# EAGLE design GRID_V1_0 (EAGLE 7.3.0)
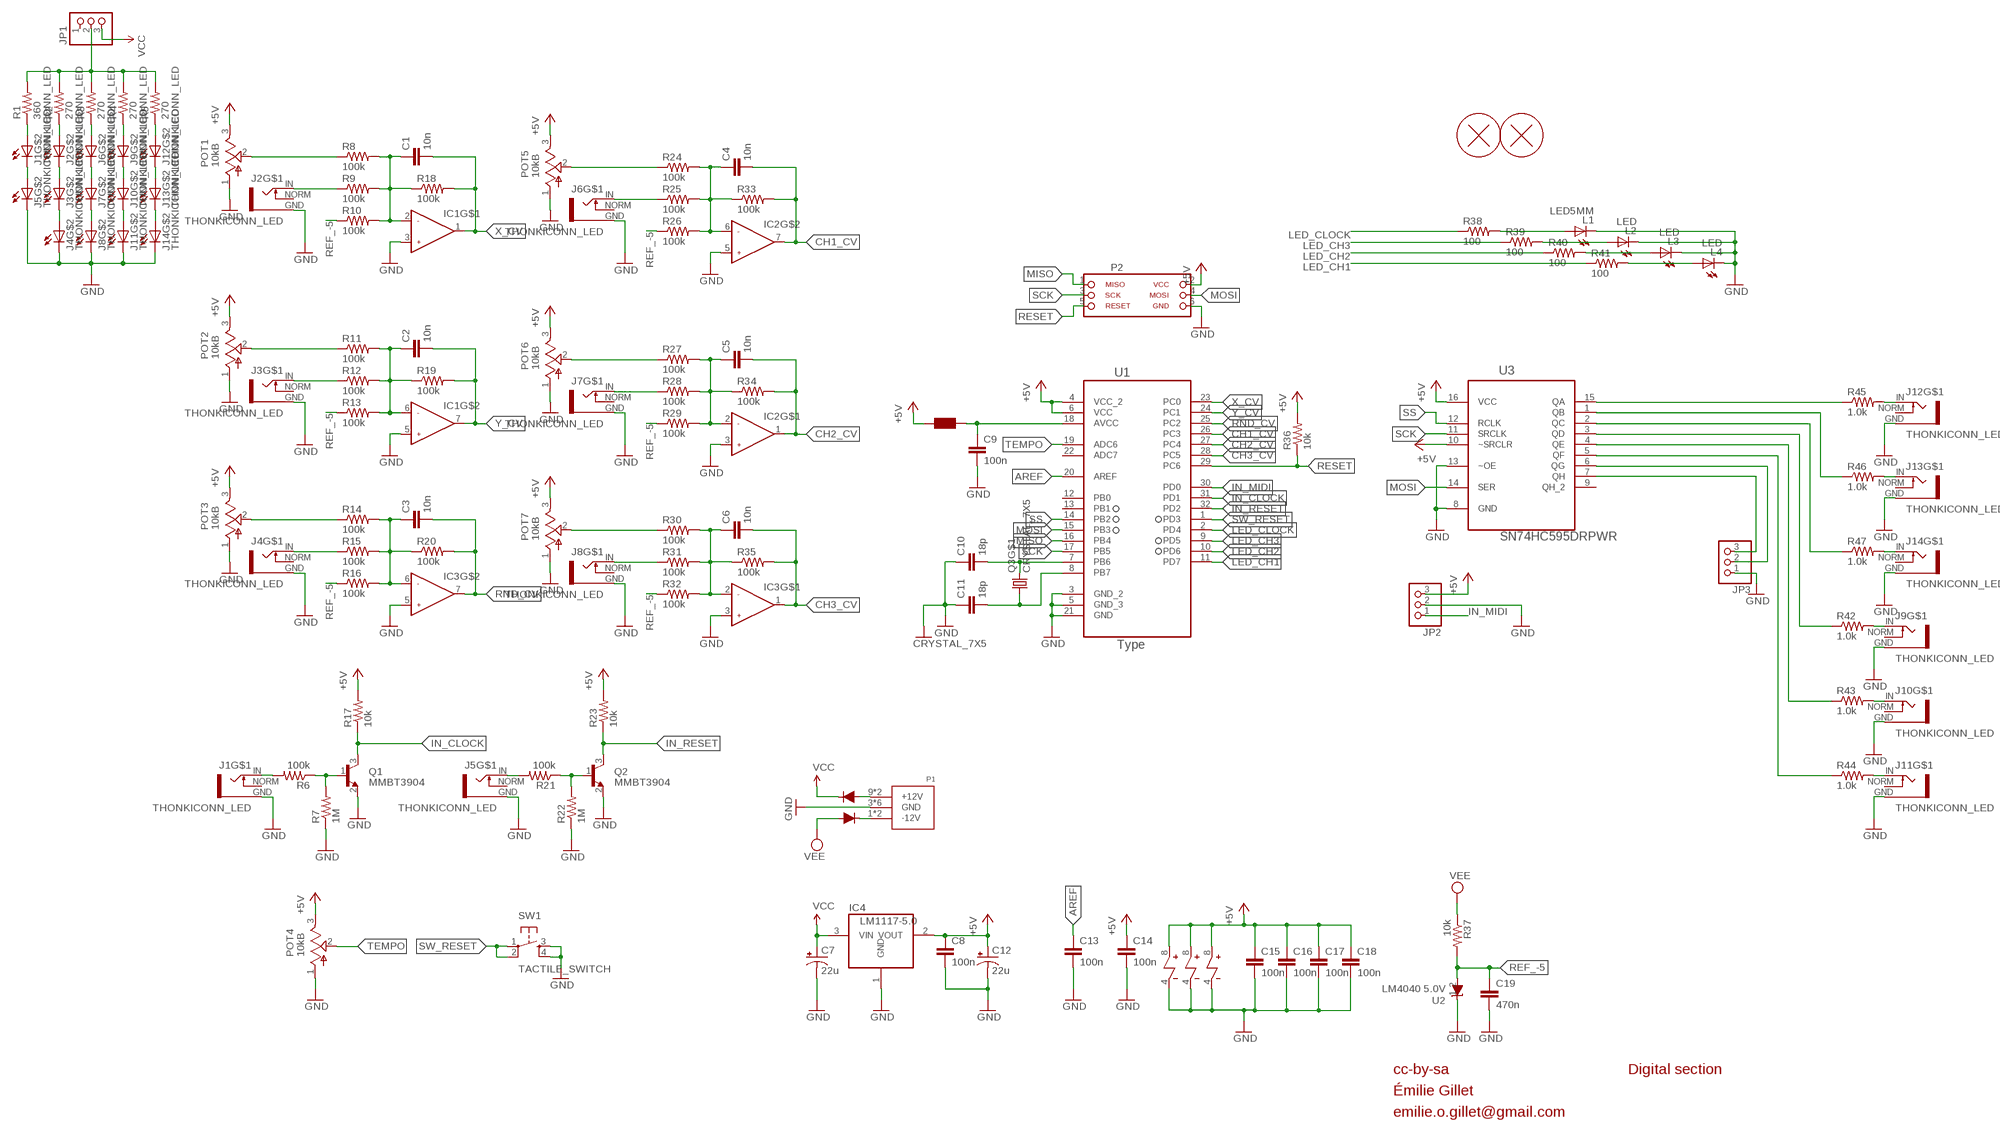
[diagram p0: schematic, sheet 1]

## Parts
C1  10n  CAPACITOR  [RESISTOR_0603]
C2  10n  CAPACITOR  [RESISTOR_0603]
C3  10n  CAPACITOR  [RESISTOR_0603]
C4  10n  CAPACITOR  [RESISTOR_0603]
C5  10n  CAPACITOR  [RESISTOR_0603]
C6  10n  CAPACITOR  [RESISTOR_0603]
C7  22u  CAP_POLC  [PANASONIC_C]
C8  100n  CAPACITOR  [RESISTOR_0603]
C9  100n  CAPACITOR  [RESISTOR_0603]
C10  18p  CAPACITOR  [RESISTOR_0603]
C11  18p  CAPACITOR  [RESISTOR_0603]
C12  22u  CAP_POLC  [PANASONIC_C]
C13  100n  CAPACITOR  [RESISTOR_0603]
C14  100n  CAPACITOR  [RESISTOR_0603]
C15  100n  CAPACITOR  [RESISTOR_0603]
C16  100n  CAPACITOR  [RESISTOR_0603]
C17  100n  CAPACITOR  [RESISTOR_0603]
C18  100n  CAPACITOR  [RESISTOR_0603]
C19  470n  CAPACITOR  [RESISTOR_0603]
D1  1N5819HW  DIODE  [SOD123]
D2  1N5819HW  DIODE  [SOD123]
F1  FERRITE-BEAD  [RESISTOR_0603]
H1  PCB_SCREW  [PCB_SCREW]
H2  PCB_SCREW  [PCB_SCREW]
IC1  OPAMP_DUAL  [SOIC8]
IC2  OPAMP_DUAL  [SOIC8]
IC3  OPAMP_DUAL  [SOIC8]
IC4  LM1117-5.0  REG1117  [SOT223]
J1  THONKICONN_LED  [LED_JACK]
J2  THONKICONN_LED  [LED_JACK]
J3  THONKICONN_LED  [LED_JACK]
J4  THONKICONN_LED  [LED_JACK]
J5  THONKICONN_LED  [LED_JACK]
J6  THONKICONN_LED  [LED_JACK]
J7  THONKICONN_LED  [LED_JACK]
J8  THONKICONN_LED  [LED_JACK]
J9  THONKICONN_LED  [LED_JACK]
J10  THONKICONN_LED  [LED_JACK]
J11  THONKICONN_LED  [LED_JACK]
J12  THONKICONN_LED  [LED_JACK]
J13  THONKICONN_LED  [LED_JACK]
J14  THONKICONN_LED  [LED_JACK]
JP1  PINHD-1X3  [1X03]
JP2  PINHD-1X3  [1X03]
JP3  PINHD-1X3  [1X03]
L1  LED5MM  [LED_5MM]
L2  LED  [LED_3MM]
L3  LED  [LED_3MM]
L4  LED  [LED_3MM]
P1  POWER_SIMPLE10  [POWER_10]
P2  PINHD-SPI  [2X03]
POT1  10kB  POT_VERTICAL  [ALPS_POT_VERTICAL]
POT2  10kB  POT_VERTICAL  [ALPS_POT_VERTICAL]
POT3  10kB  POT_VERTICAL  [ALPS_POT_VERTICAL]
POT4  10kB  POT_VERTICAL  [ALPS_POT_VERTICAL]
POT5  10kB  POT_VERTICAL  [ALPS_POT_VERTICAL]
POT6  10kB  POT_VERTICAL  [ALPS_POT_VERTICAL]
POT7  10kB  POT_VERTICAL  [ALPS_POT_VERTICAL]
Q1  MMBT3904  MMBT3904SOT23  [SOT23]
Q2  MMBT3904  MMBT3904SOT23  [SOT23]
Q3  CRYSTAL_7X5  [7X5_CRYSTAL]
R1  360  RESISTOR  [RESISTOR_0603]
R2  270  RESISTOR  [RESISTOR_0603]
R3  270  RESISTOR  [RESISTOR_0603]
R4  270  RESISTOR  [RESISTOR_0603]
R5  270  RESISTOR  [RESISTOR_0603]
R6  100k  RESISTOR  [RESISTOR_0603]
R7  1M  RESISTOR  [RESISTOR_0603]
R8  100k  RESISTOR  [RESISTOR_0603]
R9  100k  RESISTOR  [RESISTOR_0603]
R10  100k  RESISTOR  [RESISTOR_0603]
R11  100k  RESISTOR  [RESISTOR_0603]
R12  100k  RESISTOR  [RESISTOR_0603]
R13  100k  RESISTOR  [RESISTOR_0603]
R14  100k  RESISTOR  [RESISTOR_0603]
R15  100k  RESISTOR  [RESISTOR_0603]
R16  100k  RESISTOR  [RESISTOR_0603]
R17  10k  RESISTOR  [RESISTOR_0603]
R18  100k  RESISTOR  [RESISTOR_0603]
R19  100k  RESISTOR  [RESISTOR_0603]
R20  100k  RESISTOR  [RESISTOR_0603]
R21  100k  RESISTOR  [RESISTOR_0603]
R22  1M  RESISTOR  [RESISTOR_0603]
R23  10k  RESISTOR  [RESISTOR_0603]
R24  100k  RESISTOR  [RESISTOR_0603]
R25  100k  RESISTOR  [RESISTOR_0603]
R26  100k  RESISTOR  [RESISTOR_0603]
R27  100k  RESISTOR  [RESISTOR_0603]
R28  100k  RESISTOR  [RESISTOR_0603]
R29  100k  RESISTOR  [RESISTOR_0603]
R30  100k  RESISTOR  [RESISTOR_0603]
R31  100k  RESISTOR  [RESISTOR_0603]
R32  100k  RESISTOR  [RESISTOR_0603]
R33  100k  RESISTOR  [RESISTOR_0603]
R34  100k  RESISTOR  [RESISTOR_0603]
R35  100k  RESISTOR  [RESISTOR_0603]
R36  10k  RESISTOR  [RESISTOR_0603]
R37  10k  RESISTOR  [RESISTOR_0603]
R38  100  RESISTOR  [RESISTOR_0603]
R39  100  RESISTOR  [RESISTOR_0603]
R40  100  RESISTOR  [RESISTOR_0603]
R41  100  RESISTOR  [RESISTOR_0603]
R42  1.0k  RESISTOR  [RESISTOR_0603]
R43  1.0k  RESISTOR  [RESISTOR_0603]
R44  1.0k  RESISTOR  [RESISTOR_0603]
R45  1.0k  RESISTOR  [RESISTOR_0603]
R46  1.0k  RESISTOR  [RESISTOR_0603]
R47  1.0k  RESISTOR  [RESISTOR_0603]
SW1  TACTILE_SWITCH  [TACTILE-PTH]
U1  ATMEGA328P-AU  [QFP80P900X900X120-32N]
U2  LM4040 5.0V  LM4040SOT23  [SOT23]
U3  SN74HC595DRPWR  [TSSOP16]

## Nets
+5V [wide]: C8.1 C12.+ C14.1 C15.1 C16.1 C17.1 C18.1 F1.2 IC1.8 IC2.8 IC3.8 IC4.2(VOUT) JP2.3 P2.2 POT1.3(B) POT2.3(B) POT3.3(B) POT4.3(B) POT5.3(B) POT6.3(B) POT7.3(B) R17.2 R23.2 R36.2 U1.4(VCC_2) U1.6(VCC) U3.10(~SRCLR) U3.16(VCC)
AREF: C13.1 U1.20(AREF)
CH1_CV: C4.2 IC2.7 R33.2 U1.26(PC3)
CH2_CV: C5.2 IC2.1 R34.2 U1.27(PC4)
CH3_CV: C6.2 IC3.1 R35.2 U1.28(PC5)
CLOCK_OUT: JP3.2 U3.6(QG)
GATE1_IN: J1.IN R6.2
GATE1_LED: L1.A R38.2
GATE2_IN: J5.IN R21.2
GATE2_LED: L2.A R39.2
GATE3_LED: L3.A R40.2
GATE4_LED: L4.A R41.2
GND: C7.- C8.2 C9.2 C10.1 C11.1 C12.- C13.2 C14.2 C15.2 C16.2 C17.2 C18.2 C19.2 IC1.3 IC1.4 IC1.5 IC2.3 IC2.4 IC2.5 IC3.3 IC3.4 IC3.5 IC4.1(GND) J1.GND J2.GND J3.GND J4.C J4.GND J5.C J5.GND J6.GND J7.GND J8.C J8.GND J9.GND J10.GND J11.C J11.GND J12.GND J13.GND J14.C J14.GND JP2.2 JP3.1 L1.K(C) L2.K(C) L3.K(C) L4.K(C) P1.3(GND) P1.4(GND) P1.5(GND) P1.6(GND) P1.7(GND) P1.8(GND) P2.6 POT1.1(A) POT2.1(A) POT3.1(A) POT4.1(A) POT5.1(A) POT6.1(A) POT7.1(A) Q1.2(E) Q2.2(E) Q3.2(GND) Q3.4(GND) R7.1 R22.1 SW1.3 SW1.4 U1.3(GND_2) U1.5(GND_3) U1.21(GND) U2.1(C) U3.8(GND) U3.13(~OE)
IN_CLOCK: Q1.3(C) R17.1 U1.31(PD1)
IN_MIDI: JP2.1 U1.30(PD0)
IN_RESET: Q2.3(C) R23.1 U1.32(PD2)
LED_CH1: R41.1 U1.11(PD7)
LED_CH2: R40.1 U1.10(PD6)
LED_CH3: R39.1 U1.9(PD5)
LED_CLOCK: R38.1 U1.2(PD4)
MISO: P2.1 U1.16(PB4)
MOSI: P2.4 U1.15(PB3) U3.14(SER)
N$1: Q1.1(B) R6.1 R7.2
N$2: Q2.1(B) R21.1 R22.2
N$3 [wide]: D1.+ P1.9(+12V) P1.10(+12V)
N$4: J11.IN R44.2
N$5: J10.IN R43.2
N$6: J9.IN R42.2
N$8: J2.C J3.A
N$9: POT1.2(W) R8.1
N$10: J2.IN R9.1
N$11: J3.C J4.A
N$12: C2.1 IC1.6 R11.2 R12.2 R13.2 R19.1
N$13: POT2.2(W) R11.1
N$14: J3.IN R12.1
N$15: C3.1 IC3.6 R14.2 R15.2 R16.2 R20.1
N$16: POT3.2(W) R14.1
N$17: J4.IN R15.1
N$18: C4.1 IC2.6 R24.2 R25.2 R26.2 R33.1
N$19: POT5.2(W) R24.1
N$20: J6.IN R25.1
N$21: C5.1 IC2.2 R27.2 R28.2 R29.2 R34.1
N$22: POT6.2(W) R27.1
N$23: J7.IN R28.1
N$24: C6.1 IC3.2 R30.2 R31.2 R32.2 R35.1
N$25: POT7.2(W) R30.1
N$26: J8.IN R31.1
N$27: R45.1 U3.15(QA)
N$28: R46.1 U3.1(QB)
N$29: C1.1 IC1.2 R8.2 R9.2 R10.2 R18.1
N$30: R47.1 U3.2(QC)
N$31: R42.1 U3.3(QD)
N$32: R43.1 U3.4(QE)
N$33: R44.1 U3.5(QF)
N$34: J12.IN R45.2
N$35: J13.IN R46.2
N$36: J14.IN R47.2
N$37: J7.C J8.A
N$38: J6.C J7.A
N$39: C9.1 F1.1 U1.18(AVCC)
N$40: J9.C J10.A
N$41: J10.C J11.A
N$42: J12.C J13.A
N$43: J13.C J14.A
N$44: J12.A R5.1
N$45: J9.A R4.1
N$46: J6.A R3.1
N$47: J2.A R2.1
N$48: J1.A R1.1
N$49: J1.C J5.A
N$50 [wide]: JP1.2 R1.2 R2.2 R3.2 R4.2 R5.2
N$51 [wide]: D2.- P1.1(-12V) P1.2(-12V)
N$82: C11.2 Q3.1 U1.8(PB7)
N$83: C10.2 Q3.3 U1.7(PB6)
RANDOM_GATE: JP3.3 U3.7(QH)
REF_-5: C19.1 R10.1 R13.1 R16.1 R26.1 R29.1 R32.1 R37.2 U2.2(A)
RESET: P2.5 R36.1 U1.29(PC6)
RND_CV: C3.2 IC3.7 R20.2 U1.25(PC2)
SCK: P2.3 U1.17(PB5) U3.11(SRCLK)
SS: U1.14(PB2) U3.12(RCLK)
SW_RESET: SW1.1 SW1.2 U1.1(PD3)
TEMPO: POT4.2(W) U1.19(ADC6)
VCC [wide]: C7.+ D1.- IC4.3(VIN) JP1.3
VEE [wide]: D2.+ R37.1
X_CV: C1.2 IC1.1 R18.2 U1.23(PC0)
Y_CV: C2.2 IC1.7 R19.2 U1.24(PC1)
Unconnected: J1.NORM J2.NORM J3.NORM J4.NORM J5.NORM J6.NORM J7.NORM J8.NORM J9.NORM J10.NORM J11.NORM J12.NORM J13.NORM J14.NORM JP1.1 U1.12(PB0) U1.13(PB1) U1.22(ADC7) U3.9(QH_2)

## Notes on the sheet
- cc-by-sa | Digital section
- Émilie Gillet
- emilie.o.gillet@gmail.com

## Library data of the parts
C1-C6 C8-C11 C13-C19 = parts_aman:CAPACITOR
C7 C12 = parts_aman:CAP_POL
D1 D2 = parts_aman:DIODE
F1 = parts_aman:FERRITE-BEAD
H1 H2 = parts_aman:PCB_SCREW
IC1-IC3 = parts_aman:OPAMP_DUAL
IC4 = og-vreg:REG1117: 800mA and 1A Low Dropout (LDO) Positive Regulator 1.8V, 2.5V, 2.85V, 3.3V, 5V, and Adj
J1-J14 = parts_aman:THONKICONN_LED
JP1-JP3 = parts_aman:PINHD-1X3: PIN HEADER
L1-L4 = parts_aman:LED
P1 = parts_aman:POWER_SIMPLE
P2 = parts_aman:PINHD-SPI: PIN HEADER
POT1-POT7 = parts_aman:POT_VERTICAL
Q1 Q2 = parts_aman:MMBT3904
Q3 = parts_aman:CRYSTAL_7X5
R1-R47 = parts_aman:RESISTOR
SW1 = parts_aman:TACTILE_SWITCH
U1 = parts_aman:ATMEGA328P-AU; DESCRIPTION: 8-bit Microcontroller with In-System Programmable Flash; MPN: ATMEGA328P-AU; OC_FARNELL: 1715486; OC_NEWARK: 14R4631; PACKAGE: TQFP-32; SUPPLIER: Atmel
U2 = parts_aman:LM4040
U3 = parts_aman:SN74HC595DR: 8-BIT SHIFT REGISTERS WITH 3-STATE OUTPUT REGISTERS

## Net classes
0 default: width 0.152 mm, drill 0.305 mm, clearance 0.152 mm
1 wide: width 0.305 mm, drill 0.305 mm, clearance 0.152 mm

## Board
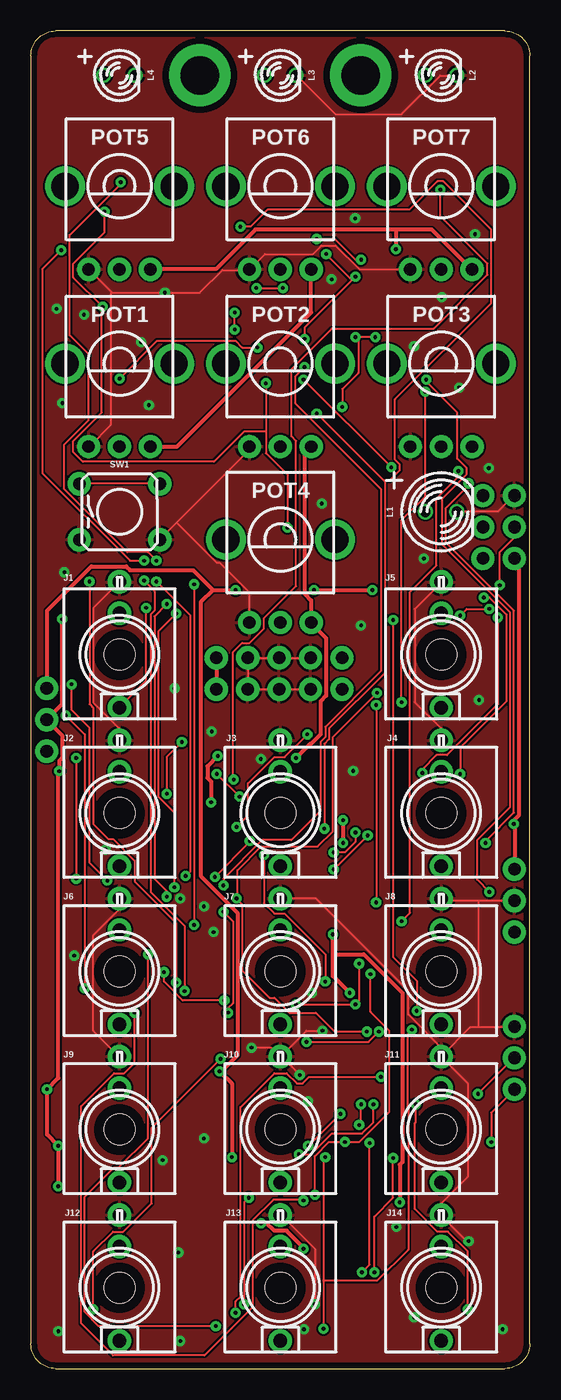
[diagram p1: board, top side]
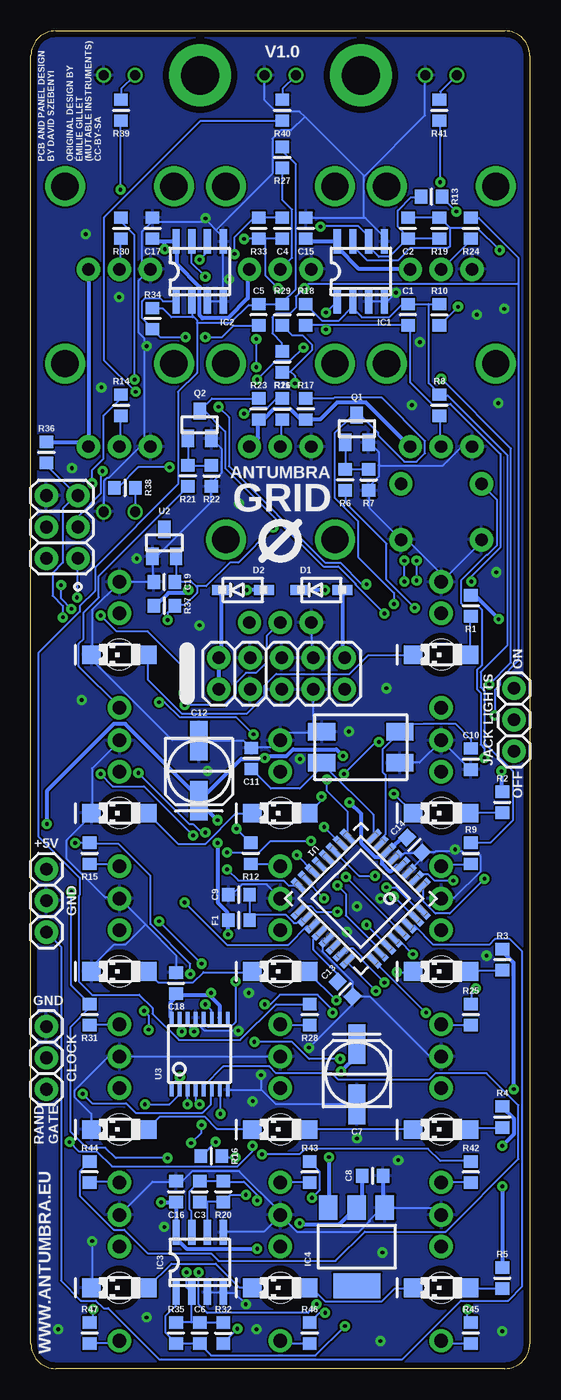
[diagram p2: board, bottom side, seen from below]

Size 40.3 x 108 mm. Coordinates in mm from the lower left corner, seen from the top.
Outline: 2,0 38.3,0 arc90 40.3,2 40.3,106 arc90 38.3,108 2,108 arc90 0,106 0,2 arc90 2,0
Copper layers (1*16): Top 0.035mm / dielectric 1.5mm / Bottom 0.035mm
Design rules "PCBCart-Standard": minimum track width 6mil, minimum drill 12mil, track to track 6mil, track to pad 6mil, pad to pad 6mil, via to via 6mil, smd to smd 6mil, copper to edge 20mil, drill to drill 8mil, minimum pad ring 8mil, minimum via ring 10mil, stop-mask expansion 3mil, vias tented up to drill 25mil, thermal gap 8mil

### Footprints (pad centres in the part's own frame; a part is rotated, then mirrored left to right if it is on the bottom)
RESISTOR_0603 = smd 1 x 1.1: 1 -0.85,0; 2 0.85,0
PANASONIC_C = smd 3.2 x 1.4: + 2.378,0; - -2.478,0
SOD123 = smd 1.6 x 0.8: + 1.7,0; - -1.7,0
PCB_SCREW = drill 3.1 pad 5: P$1 0,0
SOIC8 = smd 0.6 x 2: 1 -1.905,-2.419; 2 -0.635,-2.419; 3 0.635,-2.419; 4 1.905,-2.419; 5 1.905,2.42; 6 0.635,2.42; 7 -0.635,2.42; 8 -1.905,2.42
SOT223 = smd 1.499 x 2.007: 1 -2.261,-3.15; 2 0.025,-3.15; 3 2.311,-3.15 | smd 3.81 x 2.007: 4 0,3.15
LED_JACK = smd 1.5 x 1.5 bottom: A 2.266,0; C -2.266,0 | drill 1.1 pad 1.88: GND 0,-5.88; IN 0,4.28; NORM 0,-3.34 | hole 2.5: 0,0
1X03 = drill 1.016 pad 1.88: 1 -2.54,0; 2 0,0; 3 2.54,0
LED_5MM = drill 0.813: A -1.27,0; K 1.27,0
LED_3MM = drill 0.813: A -1.27,0; K 1.27,0
POWER_10 = drill 1.016 pad 1.88: 1 -5.08,-1.27; 2 -5.08,1.27; 3 -2.54,-1.27; 4 -2.54,1.27; 5 0,-1.27; 6 0,1.27; 7 2.54,-1.27; 8 2.54,1.27; 9 5.08,-1.27; 10 5.08,1.27
2X03 = drill 1.016 pad 1.88: 1 -2.54,-1.27; 2 -2.54,1.27; 3 0,-1.27; 4 0,1.27; 5 2.54,-1.27; 6 2.54,1.27
ALPS_POT_VERTICAL = drill 1 pad 1.88: 1 -2.5,-6.7; 2 0,-6.7; 3 2.5,-6.7 | drill 2.2 pad 3.175: P$4 4.4,0; P$5 -4.4,0
SOT23 = smd 1 x 1.4: 1 -0.95,-1.1; 2 0.95,-1.1; 3 0,1.1
7X5_CRYSTAL = smd 2.2 x 1.4: 1 -3.15,-1.25; 2 -3.15,1.25; 3 3.15,1.25; 4 3.15,-1.25
TACTILE-PTH = drill 1.016 pad 1.88: 1 -3.251,2.261; 2 3.251,2.261; 3 -3.251,-2.261; 4 3.251,-2.261
QFP80P900X900X120-32N = smd 1.473 x 0.508: 1 -4.242,2.794; 2 -4.242,2.007; 3 -4.242,1.194; 4 -4.242,0.406; 5 -4.242,-0.406; 6 -4.242,-1.194; 7 -4.242,-2.007; 8 -4.242,-2.794; 17 4.242,-2.794; 18 4.242,-2.007; 19 4.242,-1.194; 20 4.242,-0.406; 21 4.242,0.406; 22 4.242,1.194; 23 4.242,2.007; 24 4.242,2.794 | smd 0.508 x 1.473: 9 -2.794,-4.242; 10 -2.007,-4.242; 11 -1.194,-4.242; 12 -0.406,-4.242; 13 0.406,-4.242; 14 1.194,-4.242; 15 2.007,-4.242; 16 2.794,-4.242; 25 2.794,4.242; 26 2.007,4.242; 27 1.194,4.242; 28 0.406,4.242; 29 -0.406,4.242; 30 -1.194,4.242; 31 -2.007,4.242; 32 -2.794,4.242
TSSOP16 = smd 0.305 x 0.991: 1 -2.275,-2.918; 2 -1.625,-2.918; 3 -0.975,-2.918; 4 -0.325,-2.918; 5 0.325,-2.918; 6 0.975,-2.918; 7 1.625,-2.918; 8 2.275,-2.918; 9 2.275,2.918; 10 1.625,2.918; 11 0.975,2.918; 12 0.325,2.918; 13 -0.325,2.918; 14 -0.975,2.918; 15 -1.625,2.918; 16 -2.275,2.918

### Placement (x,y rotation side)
C1  9.84,85.09 270 bottom
C2  9.84,92.08 90 bottom
C3  26.67,14.29 90 bottom
C4  20,92.08 90 bottom
C5  21.91,85.09 270 bottom
C6  26.67,2.86 270 bottom
C7  13.97,23.81 90 bottom
C8  12.7,15.56 0 bottom
C9  23.5,38.26 180 bottom
C10  4.76,49.21 90 bottom
C11  22.49,49.26 270 bottom
C12  26.73,48.21 270 bottom
C13  14.92,30.64 315 bottom
C14  9.32,42.27 315 bottom
C15  18.1,92.08 90 bottom
C16  28.57,14.29 90 bottom
C17  30.48,92.08 90 bottom
C18  28.57,31.11 90 bottom
C19  29.53,63.5 180 bottom
D1  16.83,62.87 0 bottom
D2  23.18,62.87 0 bottom
F1  23.5,36.2 180 bottom
H1  13.64,104.42 0 top
H2  26.64,104.42 0 top
IC1  13.65,88.58 0 bottom
IC2  26.67,88.58 0 bottom
IC3  26.67,8.57 0 bottom
IC4  13.97,9.84 180 bottom
J1  7.16,57.64 180 top
J2  7.16,44.85 180 top
J3  20.15,44.85 180 top
J4  33.15,44.85 180 top
J5  33.15,57.64 180 top
J6  7.16,32.07 180 top
J7  20.15,32.07 180 top
J8  33.15,32.07 180 top
J9  7.16,19.31 180 top
J10  20.15,19.31 180 top
J11  33.15,19.31 180 top
J12  7.16,6.52 180 top
J13  20.15,6.52 180 top
J14  33.15,6.52 180 top
JP1  1.27,52.39 90 bottom
JP2  39.05,37.78 90 bottom
JP3  39.05,25.08 270 bottom
L1  33.15,69.18 0 top
L2  33.15,104.42 0 top
L3  20.15,104.42 0 top
L4  7.16,104.42 0 top
P1  20.05,56.11 0 bottom
P2  37.78,67.94 90 bottom
POT1  7.16,81.14 0 top
POT2  20.15,81.14 0 top
POT3  33.15,81.14 0 top
POT4  20.15,66.94 0 top
POT5  7.16,95.46 0 top
POT6  20.15,95.46 0 top
POT7  33.15,95.46 0 top
Q1  13.97,75.88 0 bottom
Q2  26.67,76.2 0 bottom
Q3  13.65,50.16 0 bottom
R1  4.76,61.59 90 bottom
R2  2.22,45.72 90 bottom
R3  2.22,33.02 90 bottom
R4  2.22,20.32 90 bottom
R5  2.22,7.3 90 bottom
R6  14.92,71.75 270 bottom
R7  13.02,71.75 90 bottom
R8  7.3,77.79 90 bottom
R9  4.76,41.59 90 bottom
R10  7.3,85.09 90 bottom
R11  20,77.47 90 bottom
R12  22.54,41.59 90 bottom
R13  7.94,94.61 180 bottom
R14  33.02,77.79 90 bottom
R15  35.56,41.59 90 bottom
R16  25.72,17.14 180 bottom
R17  18.1,77.47 270 bottom
R18  18.1,85.09 270 bottom
R19  7.3,92.08 90 bottom
R20  24.77,14.29 90 bottom
R21  27.62,72.07 270 bottom
R22  25.72,72.07 90 bottom
R23  21.91,77.47 270 bottom
R24  4.76,92.08 90 bottom
R25  4.76,28.57 90 bottom
R26  20,81.28 90 bottom
R27  20,97.79 90 bottom
R28  17.78,28.57 90 bottom
R29  20,85.09 90 bottom
R30  33.02,92.08 90 bottom
R31  35.56,28.57 90 bottom
R32  24.77,2.86 90 bottom
R33  21.91,92.08 90 bottom
R34  30.48,84.77 270 bottom
R35  28.57,2.86 270 bottom
R36  39.05,73.98 90 bottom
R37  29.53,61.59 0 bottom
R38  32.7,71.12 0 bottom
R39  33.02,101.6 90 bottom
R40  20,101.6 90 bottom
R41  7.3,101.6 90 bottom
R42  4.76,15.88 270 bottom
R43  17.78,15.88 270 bottom
R44  35.56,15.88 270 bottom
R45  4.76,2.86 270 bottom
R46  17.78,2.86 270 bottom
R47  35.56,2.86 270 bottom
SW1  7.16,69.18 0 top
U1  13.65,37.94 225 bottom
U2  29.53,66.67 0 bottom
U3  26.67,25.4 0 bottom
U$1  [LOGO_3.5]  20.16,66.83 0 bottom

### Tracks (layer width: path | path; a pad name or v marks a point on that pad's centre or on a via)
+5V  (via drill 0.3)
  Top 0.305: 29.49,91.97 32.38,91.97 35.59,88.77 POT7.3 | 29.49,91.97 18.14,91.97 14.94,88.77 9.68,88.77 POT5.3 | 29.49,91.97 v29.49,90.37 | 24.38,33.45 24.38,31.7 v25.76,30.33 | 24.38,33.45 v24.38,35.05 | v29.79,13.41 29.79,16.46 30.02,16.69 30.02,30.33 26.9,33.45 24.38,33.45 | v18.59,11.73 19.05,11.73 19.66,11.12 20.65,11.12 22.02,9.75 v22.02,9.68 | 39.09,43.97 39.09,44.35 39.4,44.65 39.4,65.08 39.09,65.38 P2.2 | 39.09,43.97 39.09,40.39 JP2.3 | v14.55,45.72 14.55,47.4 14.25,47.7 14.25,48.62 v15.09,49.45 | POT2.3 22.63,74.37 22.1,73.84 22.1,62.56 22.63,62.03 22.63,60.27 POT4.3 22.71,60.12 23.85,58.98 23.85,54.33 23.39,53.87 23.39,51.21 22.63,50.44 22.55,50.44 v21.41,49.3 | v39.01,43.97 39.09,43.97 | v25.22,44.27 v25.22,42.44 | POT6.3 22.63,88.7 22.63,85.27 11.81,74.45 9.68,74.45 POT1.3
  Bottom 0.305: C14.1 10.25,42.88 U1.6 | C8.1 13.55,13.44 IC4.2 14.1,12.95 15.39,11.66 18.52,11.66 v18.59,11.73 | U3.16 29.05,28.42 29.05,29.53 28.57,30 C18.1 28.5,30.18 25.91,30.18 | 29.49,91 IC2.8 28.5,90.91 28.5,89.15 26.67,87.33 26.67,85.04 26.44,84.81 24.38,84.81 22.78,86.41 22.78,88.62 22.71,88.7 POT6.3 | 29.49,91 30.26,91 C17.1 | C15.1 17.88,91 IC1.8 15.47,90.91 15.47,90.45 13.79,88.77 9.68,88.77 POT5.3 | R36.2 39.01,74.75 35.97,74.75 35.66,74.45 POT3.3 35.89,74.83 35.59,75.13 35.59,88.7 POT7.3 | v29.49,90.37 29.49,91 | 25.91,30.18 25.07,29.34 25.07,28.35 U3.10 | v24.38,35.05 24.38,36.2 F1.2 24.46,36.27 24.46,36.88 25.22,37.64 v25.22,42.44 | v25.76,30.33 25.91,30.18 | v29.79,13.41 28.65,13.41 C16.1 IC3.8 28.5,10.9 28.5,10.44 27.74,9.68 v22.02,9.68 | U1.4 10.44,40.62 10.74,40.62 11.2,40.16 11.35,40.16 11.96,40.77 11.96,41.3 11.58,41.68 U1.6 | v14.55,45.72 13.64,44.81 13.64,42.44 12.5,41.3 12.04,41.3 U1.6 | v15.09,49.45 15.62,49.99 19.13,49.99 19.66,49.45 21.41,49.45 | 21.41,49.45 21.64,49.45 21.87,49.23 23.32,49.23 26.67,45.87 C12.+ | POT2.3 22.63,74.45 21.95,75.13 21.95,76.5 R23.2 21.87,76.66 21.49,76.66 20.65,77.5 19.36,77.5 18.52,76.66 18.14,76.66 R17.2 17.98,76.66 16.92,76.66 15.54,78.03 13.26,78.03 9.68,74.45 POT1.3 | v21.41,49.3 21.41,49.45 | v39.01,43.97 39.01,46.63 33.6,52.05 32.69,52.05 26.67,46.02 C12.+ | v25.22,44.27 26.67,45.72 C12.+
AREF
  Bottom 0.152: C13.1 15.52,31.88 17.46,33.81 17.46,34.71 U1.20
CH1_CV  (via drill 0.3)
  Top 0.152: v15.54,39.01 15.54,39.55 18.67,42.67 21.03,42.67 23.39,45.03 23.39,50.6 23.77,50.98 23.77,51.82 28.27,56.31 28.27,71.02 21.34,77.95 21.34,80.09 v22.1,80.85 | v22.1,83.13 22.1,84.05 v26.21,88.16 25.91,87.94 v23.85,89.99
  Bottom 0.152: C4.2 20.04,92.96 21.87,92.96 R33.2 21.95,92.89 22.33,92.89 23.85,91.36 v23.85,89.99 | v15.54,39.01 14.86,38.33 14.86,36.58 12.12,33.83 12.12,33.53 U1.26 | v22.1,83.13 v22.1,80.85 | v26.21,88.16 27.36,89.31 27.36,90.98 IC2.7
CH2_CV  (via drill 0.3)
  Top 0.152: v27.81,83.29 26.44,83.29 | v13.18,63.32 v13.18,35.81 | v25.15,77.65 25.15,79.1 26.44,80.39 26.44,83.29 | 26.44,83.29 v26.21,83.29
  Bottom 0.152: v26.21,83.29 24.84,83.29 23.93,84.2 21.95,84.2 C5.2 | v27.81,83.29 29.87,83.29 30.48,83.9 R34.2 30.48,83.97 31.32,84.81 31.32,86.18 31.09,86.41 29.87,86.41 29.64,86.18 28.57,86.18 IC2.1 | v13.18,35.81 11.51,34.14 U1.27 | v13.18,63.32 13.56,63.32 15.32,65.08 16.54,65.08 24.31,72.85 24.31,76.81 v25.15,77.65
CH3_CV  (via drill 0.3)
  Top 0.152: v9.45,33.45 9.45,18.59 7.09,16.23 6.71,16.23 4.34,13.87 4.34,4.57 5.49,3.43 v14.94,3.43
  Bottom 0.152: 28.57,2.06 26.67,2.06 C6.2 26.67,1.98 25.76,1.07 17.3,1.07 v14.94,3.43 | v9.45,33.45 10.59,34.59 10.9,34.59 U1.28 | IC3.1 28.57,5.11 29.41,4.27 29.41,2.9 28.57,2.06 | 28.57,2.06 R35.2
CLOCK_OUT  (via drill 0.3)
  Top 0.152: v36.12,22.17 39.01,25.07 JP3.2
  Bottom 0.152: v36.12,22.17 35.36,21.41 32.61,21.41 31.85,20.65 26.44,20.65 25.76,21.34 25.76,22.48 U3.6
GATE1_IN  (via drill 0.3)
  Top 0.152: v9.3,61.42 9.3,55.55 7.16,53.42 J1.IN
  Bottom 0.152: v9.3,61.42 11.58,63.7 11.58,66.6 14.86,69.88 14.86,70.87 R6.2
GATE1_LED
  Bottom 0.152: R38.2 31.85,71.09 31.85,69.19 L1.A
GATE2_IN
  Bottom 0.152: R21.2 27.66,71.17 34.82,64.01 34.82,62.26 36.04,61.04 36.04,58.9 36.42,58.52 36.42,56.69 33.15,53.42 J5.IN
GATE2_LED
  Bottom 0.152: R39.2 32.99,102.49 32.99,103.33 31.93,104.39 L2.A
GATE3_LED
  Bottom 0.152: R40.2 19.96,102.49 19.96,103.33 18.9,104.39 L3.A
GATE4_LED
  Bottom 0.152: R41.2 7.24,102.49 7.24,103.1 5.94,104.39 L4.A
GND  (via drill 0.3)
  Top 0.152: v35.36,10.29 35.2,10.29 33.15,12.34 J14.GND 33.15,13.34 35.28,15.47 35.28,23.01 33.15,25.15 J11.GND | v22.94,5.18 22.94,9.68 20.19,12.42 J13.GND | 36.2,37.8 33.3,37.8 J8.GND | 36.2,37.8 39.01,37.8 JP2.2 | J6.GND 7.09,37.95 7.09,37.03 5.03,34.98 5.03,27.28 7.09,25.22 J9.GND | v23.55,27.28 22.25,27.28 20.19,25.22 | 36.2,27.58 35.51,27.58 33.15,25.22 J11.GND | 36.2,27.58 39.01,27.58 JP3.1 | J7.GND 20.19,37.95 23.01,37.95 30.48,30.48 30.48,28.57 33.45,25.6 J11.GND | 20.19,25.22 v21.72,23.7 | 20.19,25.22 J10.GND 20.12,25.22 19.43,25.91 v17.83,25.91 | 36.2,27.58 36.2,37.8 | L1.K 34.44,69.19 37.72,69.19 39.01,70.48 P2.6 | L2.K 34.37,104.39 33.07,104.39 29.95,101.27 24.61,101.27 21.49,104.39 L3.K | J2.GND 7.09,50.75 7.09,51.74 5.03,53.8 5.03,61.42 7.09,63.48 J1.GND | P1.3 22.55,54.86 20.12,54.86 P1.5 20.04,54.86 17.6,54.86 P1.7 17.53,54.86 17.53,57.38 P1.8 17.6,57.38 P1.6 20.12,57.38 22.55,57.38 P1.4 | 6.51,86.91 4.72,88.7 POT5.1 | 6.51,86.91 6.55,86.87 v10.82,86.87 13.64,86.87 15.47,88.7 17.6,88.7 POT6.1 17.68,88.77 18.9,89.99 22.78,89.99 23.47,90.68 24.61,90.68 26.52,88.77 30.63,88.77 POT7.1 | 11.77,68.31 10.44,66.98 SW1.4 | 11.77,68.31 17.6,74.14 17.6,74.37 POT2.1 | 6.51,86.91 6.48,86.87 6.48,76.2 4.72,74.45 POT1.1 | 11.77,68.31 15.01,65.08 15.24,65.08 17.6,62.71 17.6,60.27 POT4.1 | J4.GND 33.15,51.66 31.01,53.8 31.01,61.34 33.15,63.48 J5.GND
  Bottom 0.152: 11.85,13.13 IC4.1 | J14.GND 33.15,12.42 30.48,15.09 28.57,15.09 C16.2 28.57,15.16 28.04,15.16 27.28,15.93 23.47,15.93 20.19,12.65 20.19,12.42 J13.GND | v35.36,10.29 35.36,6.55 J14.C | IC4.1 11.66,12.95 7.7,12.95 7.16,12.42 J12.GND | IC3.3 25.98,6.17 24.77,6.17 IC3.4 24.77,6.1 23.85,6.1 v22.94,5.18 | IC3.5 24.77,11.05 21.49,11.05 20.19,12.34 J13.GND | IC4.1 11.89,13.03 12.95,11.96 12.95,11.89 13.79,11.05 18.82,11.05 20.12,12.34 J13.GND | J4.GND 33.15,50.67 35.36,48.46 35.36,44.88 J4.C 35.43,44.81 35.43,44.65 37.41,42.67 37.41,41.15 34.29,38.02 33.15,38.02 J8.GND 31.05,35.85 | C18.2 28.57,33.38 31.05,35.85 | 31.05,35.85 32.69,34.21 33.6,34.21 35.36,32.46 35.36,32.08 J8.C | C14.2 8.76,41.6 8.76,41.15 9.75,40.16 U1.3 | U1.5 10.9,41.3 10.44,41.3 10.13,41.6 8.84,41.6 C14.2 | C14.2 8.69,41.68 7.7,41.68 7.62,41.76 5.49,41.76 5.26,41.53 4.12,41.53 3.96,41.38 3.96,40.16 6.1,38.02 7.09,38.02 J6.GND | C13.2 14.33,30.1 14.33,31.24 16.76,33.68 16.76,34.21 16.38,34.59 U1.21 | C13.2 14.25,30.02 12.88,30.02 8.08,25.22 7.16,25.22 J9.GND | 21.72,22.48 21.64,22.48 20.5,21.34 14.02,21.34 C7.- | 21.72,22.48 24.38,22.48 U3.8 | v23.55,27.28 26.29,27.28 26.98,27.96 26.98,28.27 U3.13 | C9.2 24.31,38.33 24,38.33 23.24,39.09 21.26,39.09 20.19,38.02 J7.GND | J11.C 35.43,19.36 35.43,20.57 36.8,21.95 36.8,22.4 34.06,25.15 33.15,25.15 J11.GND 33.15,25.22 20.19,25.22 J10.GND | v21.72,23.7 21.72,22.48 | v17.83,25.91 14.25,29.49 14.25,29.95 C13.2 | 31.17,74.37 31.55,74.37 33.98,71.93 34.14,71.93 34.37,71.7 34.37,69.19 L1.K | 31.17,74.37 30.71,74.37 POT3.1 31.17,74.37 | 24.77,86.18 25.98,86.18 IC2.3
  Bottom 0.152: 24.77,86.18 IC2.5 24.77,91.36 25.34,91.94 | 24.77,86.18 IC2.4 | 25.34,91.94 25.98,92.58 30.48,92.58 C17.2 30.48,92.66 31.32,91.82 31.32,89.38 30.71,88.77 POT7.1 30.71,88.7 31.62,87.78 31.62,83.67 31.17,83.21 31.17,74.37 | 13.41,92.89 13.26,92.89 11.81,91.44 11.81,91.06 IC1.5 | 13.41,92.89 18.06,92.89 C15.2 | 13.37,96.28 13.41,96.24 13.41,92.89 | 13.37,96.28 8.46,101.19 8.46,104.39 L4.K | 13.37,96.28 18.17,101.08 | 18.17,101.08 18.59,101.5 20.5,101.5 21.41,102.41 21.41,104.39 L3.K | 25.34,91.94 20.8,96.47 20.8,99.29 20.12,99.97 19.28,99.97 18.17,101.08 | C10.1 4.8,48.39 7.09,50.67 J2.GND 7.16,50.67 8.91,48.92 10.44,48.92 Q3.4 | SW1.3 3.96,66.9 3.96,66.67 7.09,63.55 J1.GND 6.86,63.86 9.91,66.9 10.36,66.9 SW1.4 10.44,66.98 12.95,69.49 12.95,70.87 R7.1 12.95,70.94 12.95,71.25 12.19,72.01 12.19,72.92 | Q2.2 25.68,75.06 24.92,74.3 24.92,72.31 25.68,71.55 25.68,71.25 R22.1 25.76,71.17 25.76,69.95 30.1,65.61 30.4,65.61 U2.1 30.48,63.6 C19.2 30.48,63.55 33.15,63.55 J5.GND 33.15,63.48 35.36,61.27 35.36,57.68 J5.C 35.36,57.61 35.36,57.23 28.88,50.75 26.75,50.75 C12.- 26.67,50.67 23.09,50.67 22.55,50.14 C11.1 22.48,50.14 20.73,50.14 20.19,50.67 J3.GND 20.12,50.75 19.51,51.36 17.53,51.36 | 17.53,51.36 16.84,51.36 Q3.2 17.53,51.36 | POT4.1 17.6,60.2 17.6,57.53 17.53,57.45 P1.8 | 17.53,51.36 17.53,54.79 P1.7 | IC1.3 12.95,86.18 11.81,86.18 IC1.4 11.73,86.18 11.51,86.18 v10.82,86.87 | 12.19,72.92 12.19,73.99 12.95,74.75 Q1.2 | 12.19,72.92 7.01,72.92 5.56,74.37 4.72,74.37 POT1.1
  Bottom 0.305: C8.2 11.85,13.13
  other vias: 4.29,85.09 2.06,85.57 9.53,77.79 23.5,69.85 34.61,79.22 30.96,82.55 33.18,86.52 35.88,91.6 2.54,77.95 11.59,54.93 36.2,53.98 26.67,60.01 26.04,48.26 2.22,3.02 10.64,16.83 22.38,21.59 30.96,4.13 38.1,3.17 22.07,3.17 12.06,2.22 11.91,9.37 29.53,11.43 13.97,18.57 22.7,30.32 14.76,35.24 12.06,37.94 13.97,37.31 14.61,51.44 18.57,49.21 2.7,64.29 36.99,72.71 8.89,82.87 26.19,92.87 24.29,87.95 31.75,65.41 3.49,33.34 6.03,41.91
  pour Top: 0,0 40.32,0 40.32,107.95 0,107.95
  pour Bottom: 0,0 40.32,0 40.32,107.95 0,107.95
IN_CLOCK  (via drill 0.3)
  Top 0.152: v10.97,38.1 10.97,38.56 9.98,39.55 9.98,60.73 v10.97,61.72
  Bottom 0.152: R17.1 18.06,78.33 15.85,78.33 15.77,78.41 11.96,78.41 8.46,74.91 8.46,73.91 9.14,73.23 10.13,73.23 12.27,75.36 12.27,75.59 13.64,76.96 13.95,76.96 Q1.3 14.02,76.96 14.33,76.96 15.77,75.51 15.77,70.33 13.87,68.43 13.87,65.53 10.97,62.64 v10.97,61.72 | v10.97,38.1 9.3,36.42 U1.31
IN_MIDI
  Bottom 0.152: JP2.1 37.87,34.06 37.87,7.09 36.27,5.49 35.05,5.49 34.44,4.88 34.06,4.88 29.95,0.76 10.29,0.76 5.56,5.49 1.75,5.49 0.61,6.63 0.61,33.68 1.6,34.67 2.82,34.67 3.28,34.21 7.77,34.21 9.3,35.74 9.75,35.74 U1.30
IN_RESET  (via drill 0.3)
  Top 0.152: v11.58,38.86 11.58,44.88 10.29,46.18 10.29,59.51 v11.73,60.96
  Bottom 0.152: R23.1 21.95,78.33 25.68,78.33 26.67,77.34 Q2.3 26.44,77.5 24.61,75.67 24.61,72.69 16.69,64.77 15.47,64.77 14.1,63.4 14.1,63.32 v11.73,60.96 | v11.58,38.86 10.82,38.86 8.91,36.96 8.69,36.96 U1.32
LED_CH1  (via drill 0.3)
  Top 0.152: v7.24,95.78 7.24,95.63 3.12,91.52 3.12,83.44 4.65,81.92 4.65,76.58 2.67,74.6 2.67,71.02 7.77,65.91 9.45,65.91 v10.13,65.23 | v10.13,63.55 12.88,60.81 12.88,40.16 v12.5,39.78
  Bottom 0.152: v7.24,95.78 7.24,100.74 R41.1 | v10.13,63.55 v10.13,65.23 | v12.5,39.78 13.79,39.78 15.77,41.76 U1.11
LED_CH2  (via drill 0.3)
  Top 0.152: v31.85,78.87 31.85,70.41 29.95,68.5 v29.95,53.8 | v22.33,51.21 20.5,49.38 19.66,49.38 17.53,47.24 17.53,44.65 v16.61,43.74
  Bottom 0.152: v31.85,78.87 34.37,81.38 34.37,92.96 26.59,100.74 20.04,100.74 R40.1 | v29.95,53.8 29.49,53.8 28.27,52.58 23.7,52.58 v22.33,51.21 | v16.61,43.74 U1.10
LED_CH3  (via drill 0.3)
  Top 0.152: v33.07,95.17 33.07,93.04 36.88,89.23 36.88,88.32 32.54,83.97 24.31,83.97 21.03,80.7 21.03,75.29 21.41,74.91 21.41,63.17 18.82,60.58 18.82,59.74 17.68,58.6 17.07,58.6 16.31,57.84 16.31,47.62 v16.38,47.55
  Bottom 0.152: v33.07,95.17 33.07,100.74 R39.1 | v16.38,47.55 16.38,46.63 14.71,44.96 14.71,42.98 U1.9
LED_CLOCK  (via drill 0.3)
  Top 0.152: v22.02,79.86 v29.11,72.77 | v18.29,82.45 17.07,82.45 16.54,82.98 10.21,82.98 v7.16,79.93 | v3.28,55.24 3.28,53.19 4.72,51.74 4.72,40.84 v6.17,39.4
  Bottom 0.152: v29.11,72.77 31.62,72.77 33.22,71.17 33.53,71.17 R38.1 | v22.02,79.86 20.5,81.38 19.36,81.38 v18.29,82.45 | v7.16,79.93 1.52,74.3 1.52,57 v3.28,55.24 | v6.17,39.4 7.7,39.4 8.23,39.93 8.84,39.93 9.22,39.55 U1.2
MISO  (via drill 0.3)
  Top 0.152: v27.2,43.05 v24.46,40.31 | v34.67,48.01 34.67,50.14 38.41,53.87 38.41,60.88 37.03,62.26 v36.58,62.26
  Bottom 0.152: v24.46,40.31 23.55,39.4 19.89,39.4 19.51,39.01 18.67,39.01 U1.16 | v27.2,43.05 31.17,47.02 33.68,47.02 v34.67,48.01 | v36.58,62.26 36.58,65.38 P2.1
MOSI  (via drill 0.3)
  Top 0.152: v27.13,27.2 24.54,27.2 23.01,28.73 20.88,28.73 19.66,29.95 19.28,29.95 17.07,32.16 17.07,37.49 v16.61,37.95 16.69,37.95 16.69,40.23 18.59,42.14 23.16,42.14 24.38,43.36 24.38,50.98 v27.96,54.56 | v37.87,63.25 37.87,65.91 39.01,67.06 39.01,67.89 P2.4 | v37.03,61.34 35.2,61.34 v34.67,60.81
  Bottom 0.152: v27.13,27.2 27.58,27.66 27.58,28.27 U3.14 | v16.61,37.95 18.14,39.47 U1.15 | v37.87,63.25 37.87,62.18 v37.03,61.34 | v34.67,60.81 33.38,59.51 30.86,59.51 27.96,56.62 v27.96,54.56
N$1
  Bottom 0.152: R7.2 13.03,72.62 14.86,72.62 R6.1 14.86,72.69 14.86,74.75 Q1.1
N$2
  Bottom 0.152: R22.2 25.76,72.92 27.58,72.92 R21.1 27.58,73 27.58,75.06 Q2.1
N$3
  Top 0.305: P1.9 15.01,54.86 15.01,57.38 P1.10
  Bottom 0.305: D1.+ 15.09,62.87 15.09,57.53 15.01,57.45 P1.10
N$4
  Bottom 0.152: R44.2 35.51,15.09 33.15,15.09 J11.IN
N$5
  Bottom 0.152: R43.2 17.83,15.09 20.12,15.09 J10.IN
N$6
  Bottom 0.152: R42.2 4.8,15.09 7.09,15.09 J9.IN
N$8  (via drill 0.3)
  Top 0.152: v10.97,46.41 10.97,49.38 v12.19,50.6 | v16.84,46.18 v15.01,48.01
  Bottom 0.152: v10.97,46.41 9.45,44.88 J2.C | v12.19,50.6 12.42,50.6 v15.01,48.01 | v16.84,46.18 16.84,45.87 17.83,44.88 J3.A
N$9
  Bottom 0.152: R8.1 7.24,76.89 7.24,74.52 POT1.2
N$10
  Bottom 0.152: R9.1 4.8,40.69 7.01,40.69 7.09,40.62 J2.IN
N$11
  Bottom 0.152: J3.C 22.48,44.81 23.77,44.81 26.21,42.37 28.42,42.37 30.86,44.81 J4.A
N$12  (via drill 0.3)
  Top 0.152: v23.7,43.59 23.7,50.44 24.08,50.83 24.08,51.66 28.57,56.16 28.57,71.63 28.54,71.67 | v23.09,77.11 28.54,71.67 | v16.92,92.2 17.75,92.2 19.13,93.57 30.56,93.57 32.84,95.86 33.3,95.86 37.19,91.97 37.19,86.03 29.41,78.26 29.41,73.38 29.79,73 29.79,72.54 28.96,71.7 28.57,71.7 28.54,71.67
  Bottom 0.152: R19.1 7.32,91.29 9.83,91.29 C2.1 | R13.2 8.84,94.56 9.6,94.56 10.67,93.5 10.67,92.2 9.83,91.36 C2.1 | C2.1 9.91,91.21 11.35,89.76 12.19,89.76 12.95,90.53 12.95,90.98 IC1.6 13.03,91.06 13.03,91.44 13.87,92.28 16.84,92.28 v16.92,92.2 | v23.7,43.59 22.55,42.44 R12.2 | v23.09,77.11 22.86,77.11 22.4,77.57 21.18,77.57 20.5,78.26 20.04,78.26 R11.2
N$13
  Bottom 0.152: R11.1 20.04,76.58 20.04,74.52 20.12,74.45 POT2.2
N$14
  Bottom 0.152: R12.1 22.48,40.69 20.27,40.69 20.19,40.62 J3.IN
N$15  (via drill 0.3)
  Top 0.152: v22.94,14.02 22.94,17.14 24.08,18.29 v25.38,18.29 26.52,18.29 28.96,20.73 28.96,27.28 27.43,28.8 v27.43,31.85 | v35.36,71.48 35.36,71.32 33.53,69.49 33.53,66.67 39.01,61.19 39.01,44.88 36.73,42.6 v36.73,42.44
  Bottom 0.152: 26.06,13.49 26.67,13.49 C3.1 | 26.06,13.49 24.77,13.49 | v25.38,18.29 26.52,17.14 R16.2 | v22.94,14.02 24.23,14.02 24.77,13.49 | 24.77,13.49 R20.1 | v27.43,31.85 27.43,32.69 30.63,35.89 30.63,39.78 33.22,42.37 35.51,42.37 R15.2 35.59,42.44 v36.73,42.44 | v35.36,71.48 35.36,72.54 34.44,73.46 34.44,76.96 33.07,78.33 33.07,78.56 R14.2 | 26.06,13.49 26.06,11.05 IC3.6
N$16
  Bottom 0.152: R14.1 33.07,76.89 33.07,74.52 POT3.2
N$17
  Bottom 0.152: R15.1 35.51,40.69 33.22,40.69 33.15,40.62 J4.IN
N$18  (via drill 0.3)
  Top 0.152: v4.34,30.71 4.34,51.21 v2.82,52.73 | v18.21,87.25 v20.34,87.25 | v26.67,89.53 26.21,89.53 24.54,91.21 v23.09,91.21
  Bottom 0.152: 21.34,91.29 21.87,91.29 R33.1 21.95,91.21 v23.09,91.21 | 21.34,91.29 20.04,91.29 C4.1 | v4.34,30.71 4.72,30.33 4.72,29.49 R25.2 | v2.82,52.73 2.82,54.79 2.44,55.17 2.44,55.63 0.91,57.15 0.91,87.55 | 0.91,87.55 0.91,89.69 4.12,92.89 4.72,92.89 R24.2 | 0.91,87.55 17.91,87.55 v18.21,87.25 18.9,86.56 18.9,85.65 19.36,85.19 20.5,85.19 20.8,84.89 20.8,83.59 20.04,82.83 20.04,82.14 R26.2 | 21.34,91.29 21.34,88.24 v20.34,87.25 | v26.67,89.53 26.06,90.14 26.06,90.98 IC2.6
N$19
  Bottom 0.152: R24.1 4.8,91.21 4.8,91.06 7.09,88.77 POT5.2
N$20
  Bottom 0.152: R25.1 4.8,27.74 7.09,27.74 J6.IN
N$21
  Bottom 0.152: R27.2 19.96,98.6 19.96,98.3 18.9,97.23 18.9,87.17 20.04,86.03 R29.2 20.04,85.95 21.87,85.95 C5.1 21.95,85.88 22.71,85.88 24.16,84.43 26.9,84.43 | 26.9,84.43 26.9,84.66 27.16,84.92 | 26.9,84.43 26.9,80.39 28.42,78.87 28.42,71.4 35.13,64.69 35.13,62.79 36.35,61.57 36.35,61.11 39.7,57.76 39.7,42.98 36.35,39.62 36.35,38.25 36.42,38.18 36.42,31.24 35.36,30.18 31.55,30.18 30.48,29.11 30.48,28.65 28.35,26.52 23.39,26.52 20.5,29.41 17.83,29.41 R28.2 | 27.16,84.92 27.28,85.04 27.28,86.11 IC2.2 | R34.1 30.48,85.57 29.64,85.57 28.96,84.89 27.2,84.89 27.16,84.92
N$22
  Bottom 0.152: R27.1 19.96,96.93 19.96,94.34 19.2,93.57 19.2,89.69 20.12,88.77 POT6.2
N$23
  Bottom 0.152: R28.1 17.83,27.74 20.12,27.74 J7.IN
N$24  (via drill 0.3)
  Top 0.152: v29.26,16.99 29.26,13.79 27.74,12.27 v27.74,7.77 | v31.93,79.86 31.93,79.7 34.44,77.19 34.44,73.46 35.2,72.69 35.2,72.24 33.22,70.26 33.22,66.52 38.71,61.04 38.71,45.34 36.04,42.67 36.04,39.47 v37.03,38.48
  Bottom 0.152: 26.67,3.73 24.77,3.73 R32.2 | 26.67,3.73 27.36,3.73 | 27.36,3.73 28.57,3.73 R35.1 | 26.67,3.73 C6.1 | v29.26,16.99 33.45,16.99 34.29,17.83 35.81,17.83 37.11,19.13 37.11,27.58 35.59,29.11 35.59,29.41 R31.2 35.59,29.49 37.03,30.94 v37.03,38.48 | v27.74,7.77 27.74,6.55 27.36,6.17 IC3.2 27.36,6.1 27.36,3.73 | v31.93,79.86 31.93,91.52 32.99,92.58 32.99,92.89 R30.2
N$25
  Bottom 0.152: R30.1 33.07,91.21 33.07,88.85 33.15,88.77 POT7.2
N$26
  Bottom 0.152: R31.1 35.51,27.74 33.15,27.74 J8.IN
N$27  (via drill 0.3)
  Top 0.152: v28.12,27.2 27.28,26.36 v22.25,26.36 | v15.32,24.99 9.75,19.43 9.75,13.34 7.47,11.05 6.63,11.05 5.03,9.45 v5.03,4.8
  Bottom 0.152: v28.12,27.2 28.27,27.36 28.27,28.27 U3.15 | v22.25,26.36 19.2,26.36 17.83,24.99 v15.32,24.99 | v5.03,4.8 5.03,3.96 4.8,3.73 R45.1
N$28  (via drill 0.3)
  Top 0.152: v28.27,23.55 22.48,23.55 21.95,23.01 21.49,23.01 20.65,23.85 19.66,23.85 16.92,21.11 16.92,5.79 16.54,5.41 v16.54,4.5
  Bottom 0.152: v28.27,23.55 28.88,22.94 28.88,22.55 U3.1 | v16.54,4.5 16.99,4.5 17.75,3.73 R46.1
N$29
  Bottom 0.152: 8.15,85.95 9.83,85.95 C1.1 9.91,85.88 10.36,85.88 11.35,84.89 13.56,84.89 14.33,85.65 IC1.2 14.33,86.11 14.33,85.72 15.47,84.58 16.76,84.58 18.06,85.88 R18.1 | 8.15,85.95 7.32,85.95 R10.2 | R9.2 4.72,42.44 3.2,42.44 1.37,44.27 1.37,48.23 3.66,50.52 3.66,54.71 3.96,55.02 3.96,56.24 1.83,58.37 1.83,73.76 6.63,78.56 7.24,78.56 R8.2 7.32,78.72 8.15,79.55 8.15,85.95
N$30  (via drill 0.3)
  Top 0.152: v31.09,21.34 31.09,19.89 31.01,19.81 31.01,12.88 32.84,11.05 33.68,11.05 35.28,9.45 v35.28,4.8
  Bottom 0.152: v31.09,21.34 29.11,21.34 28.35,22.1 28.35,22.48 U3.2 | v35.28,4.8 35.28,3.96 35.51,3.73 R47.1
N$31  (via drill 0.3)
  Top 0.152: v27.66,21.34 27.66,19.89 26.75,18.97 24.31,18.97 22.63,17.3 v21.64,17.3
  Bottom 0.152: v27.66,21.34 27.66,22.48 U3.3 | v21.64,17.3 18.59,17.3 18.14,17.75 8.23,17.75 7.24,16.76 4.8,16.76 R42.1
N$32  (via drill 0.3)
  Top 0.152: v26.67,21.34 26.67,19.81 v26.52,19.66 | v27.36,18.21 27.36,8.38 v26.75,7.77 | v17.22,5.18 17.22,13.41 v17.6,13.79
  Bottom 0.152: v26.67,21.34 26.98,21.64 26.98,22.48 U3.4 | v26.52,19.66 26.52,19.05 v27.36,18.21 | v26.75,7.77 26.75,5.18 26.06,4.5 17.91,4.5 v17.22,5.18 | v17.6,13.79 16.99,14.4 16.99,15.93 17.75,16.69 R43.1
N$33
  Bottom 0.152: U3.5 26.29,22.55 26.29,22.86 24.77,24.38 21.03,24.38 20.5,23.85 16,23.85 15.47,23.32 8.15,23.32 7.62,23.85 3.5,23.85 0.91,21.26 0.91,16.92 6.78,11.05 13.34,11.05 15.7,8.69 25.15,8.69 25.76,9.3 30.86,9.3 32.77,11.2 33.6,11.2 36.35,13.95 36.35,15.93 35.59,16.69 R44.1
N$34
  Bottom 0.152: R45.2 4.8,2.06 6.93,2.06 7.09,2.21 J12.IN
N$35
  Bottom 0.152: R46.2 17.83,2.06 19.96,2.06 20.12,2.21 J13.IN
N$36
  Bottom 0.152: R47.2 35.51,2.06 33.3,2.06 33.15,2.21 J14.IN
N$37
  Bottom 0.152: J7.C 22.48,32 26.36,32 27.2,31.17 30.02,31.17 30.86,32 J8.A
N$38  (via drill 0.3)
  Top 0.152: v10.74,32 10.74,31.24 12.27,29.72 v15.62,29.72
  Bottom 0.152: v10.74,32 9.45,32 J6.C | v15.62,29.72 17.91,32 J7.A
N$39
  Bottom 0.152: C9.1 F1.1 22.63,36.65 19.74,36.65 19.05,35.97 18.82,35.97 18.44,36.35 18.14,36.35 U1.18
N$40
  Bottom 0.152: J9.C 9.45,19.36 17.83,19.36 J10.A
N$41
  Bottom 0.152: J10.C 22.48,19.36 25.3,19.36 26.29,20.34 29.87,20.34 30.86,19.36 J11.A
N$42
  Bottom 0.152: J12.C 9.45,6.48 10.9,6.48 11.96,5.41 16.54,5.41 17.6,6.48 17.83,6.48 J13.A
N$43
  Bottom 0.152: J13.C 22.48,6.55 23.47,6.55 25.38,8.46 28.96,8.46 30.86,6.55 J14.A
N$44
  Bottom 0.152: R5.1 2.29,6.48 4.88,6.48 J12.A
N$45
  Bottom 0.152: R4.1 2.29,19.43 4.8,19.43 4.88,19.36 J9.A
N$46
  Bottom 0.152: R3.1 2.29,32.16 4.8,32.16 4.88,32.08 J6.A
N$47
  Bottom 0.152: R2.1 2.29,44.88 4.88,44.88 J2.A
N$48
  Bottom 0.152: R1.1 4.8,60.73 4.8,57.76 4.88,57.68 J1.A
N$49
  Bottom 0.152: J1.C 9.45,57.61 13.03,57.61 14.55,56.08 20.5,56.08 21.41,55.17 21.41,54.33 22.86,52.88 28.12,52.88 30.86,55.63 30.86,57.61 J5.A
N$50  (via drill 0.3)
  Top 0.305: v2.52,60.5 2.52,53.65 1.37,52.5 JP1.2 1.29,52.35 2.52,51.13 2.52,49.3 2.29,49.07 v2.29,48.23 2.21,48.16 2.21,23.47 v1.29,22.55 1.29,18.9 v2.21,17.98 v2.21,14.71
  Bottom 0.305: v2.29,48.23 2.29,46.63 R2.2 | v2.52,60.5 4.42,62.41 4.72,62.41 R1.2 | v2.21,14.71 R5.2 | v2.21,17.98 1.29,18.9 1.29,20.19 2.21,21.11 R4.2 | v1.29,22.55 1.29,32.77 2.21,33.68 2.21,33.83 R3.2
N$51
  Bottom 0.305: D2.- 24.92,62.87 24.92,57.61 25.07,57.45 P1.2 25.15,57.23 25.15,54.86 P1.1
N$82
  Bottom 0.152: C11.2 20.91,46.83 18.57,46.83 16.81,48.6 Q3.1 16.76,48.54 16.46,48.54 12.65,44.73 12.65,42.98 U1.8
N$83
  Bottom 0.152: C10.2 4.76,50.8 6.03,52.07 8.57,52.07 10.18,52.05 Q3.3 10.52,51.36 11.89,49.99 11.89,48.16 11.66,47.93 11.66,43.13 12.04,42.75 12.04,42.37 U1.7
RANDOM_GATE  (via drill 0.3)
  Top 0.152: v22.4,17.98 v24.99,20.57 | v37.19,18.29 37.19,20.65 39.01,22.48 JP3.3
  Bottom 0.152: v24.99,20.57 24.99,22.48 U3.7 | v22.4,17.98 22.4,17.53 23.62,16.31 33.76,16.31 34.98,17.53 36.42,17.53 v37.19,18.29
REF_-5  (via drill 0.3)
  Top 0.152: 23.62,7.09 23.62,16.92 v23.77,17.07 | 23.62,7.09 v23.62,3.2 | v5.94,93.42 5.94,91.75 3.43,89.23 3.43,88.09 v5.79,85.72 5.71,85.72 5.71,77.19 3.43,74.91 3.43,73.99 4.19,73.23 14.78,73.23 17.22,75.67 18.97,75.67 | v20.73,67.89 20.73,72.16 18.97,73.91 18.97,75.67 | v18.97,79.55 18.97,75.67 | 23.62,7.09 27.96,7.09 30.48,9.6 30.48,21.03 30.4,21.11 30.4,26.98 v30.79,27.36 | v31.17,28.88 31.17,31.32 29.26,33.22 v29.26,60.43
  Bottom 0.152: U2.2 28.58,63.6 C19.1 28.57,63.55 27.36,63.55 26.94,63.13 | v23.62,3.2 24.77,2.06 R32.1 | v23.77,17.07 24.77,17.07 24.84,17.14 R16.1 | v5.94,93.42 7.09,94.56 R13.1 | v5.79,85.72 7.24,84.28 R10.1 | 26.94,63.13 26.9,63.09 26.9,62.64 27.89,61.65 28.65,61.65 R37.2 28.73,61.57 29.26,61.04 v29.26,60.43 | 19.32,80.5 17.6,82.22 17.6,82.68 18.36,83.44 19.2,83.44 19.96,84.2 R29.1 | 19.32,80.5 19.36,80.47 19.96,80.47 R26.1 | v20.73,67.89 23.55,65.08 24.23,65.08 26.14,63.17 26.9,63.17 26.94,63.13 | v18.97,79.55 18.97,80.16 19.32,80.5 | v30.79,27.36 30.79,28.5 v31.17,28.88
RESET  (via drill 0.3)
  Top 0.152: v14.86,39.7 17.68,42.52 v17.68,42.6 | v24.46,41.68 25.38,41.68 26.21,42.52 v26.21,43.28 | v31.62,48.08 31.62,48.39 32.77,49.53 33.6,49.53 37.72,53.65 v37.72,60.66
  Bottom 0.152: R36.1 39.01,73.08 39.01,72.92 36.58,70.48 P2.5 36.65,70.48 37.72,69.42 37.72,65.08 38.56,64.24 38.56,62.41 37.72,61.57 v37.72,60.66 | v14.86,39.7 10.44,35.28 U1.29 | v17.68,42.6 20.95,42.6 21.87,41.68 v24.46,41.68 | v26.21,43.28 26.52,43.28 27.2,43.97 27.51,43.97 v31.62,48.08
RND_CV  (via drill 0.3)
  Top 0.152: v8.38,28.73 8.38,24.69 7.54,23.85 6.71,23.85 4.04,21.18 4.04,3.66 6.63,1.07 14.02,1.07 17.91,4.95 17.91,11.96 19.58,13.64 21.95,13.64 v22.02,13.56
  Bottom 0.152: v8.38,28.73 12.57,32.92 U1.25 | v22.02,13.56 22.02,14.02 23.09,15.09 24.77,15.09 R20.2 24.77,15.16 26.67,15.16 C3.2 26.67,15.09 27.51,14.25 27.51,12.88 27.36,12.72 27.36,11.05 IC3.7
SCK  (via drill 0.3)
  Top 0.152: v21.41,29.41 v26.21,29.41 26.52,29.72 v26.52,32.69 | v15.93,28.73 15.93,29.11 16.31,29.49 16.31,36.12 v15.54,36.88 | v34.52,72.47 34.52,72.01 32.77,70.26 32.77,64.85 30.63,62.71 30.63,36.8 v29.95,36.12
  Bottom 0.152: v26.21,29.41 25.76,28.96 25.76,28.35 U3.11 | v21.41,29.41 20.95,29.41 20.19,30.18 17.14,30.18 15.93,28.96 v15.93,28.73 | v15.54,36.88 17.22,36.88 17.68,37.34 18.21,37.34 18.59,36.96 U1.17 | v34.52,72.47 34.67,72.31 34.67,70.64 36.5,68.81 36.5,67.97 P2.3 | v26.52,32.69 v29.95,36.12
SS  (via drill 0.3)
  Top 0.152: v23.77,31.24 23.77,33.45 20.5,36.73 19.66,36.73 18.82,37.57 v18.82,41.45
  Bottom 0.152: v23.77,31.24 23.77,27.96 24.16,27.58 25.98,27.58 26.29,27.89 26.29,28.27 U3.12 | v18.82,41.45 17.53,40.16 U1.14
SW_RESET  (via drill 0.3)
  Top 0.152: v3.66,49.3 v3.66,39.55 | SW1.2 10.36,71.48 3.96,71.48 SW1.1
  Bottom 0.152: v3.66,39.55 6.48,36.73 7.62,36.73 8.61,37.72 8.61,38.94 U1.1 | v3.66,49.3 3.66,50.06 3.96,50.37 3.96,54.56 4.27,54.86 4.27,56.39 3.89,56.77 3.89,61.27 4.27,61.65 5.41,61.65 5.56,61.8 5.56,63.63 3.5,65.68 3.43,65.68 2.67,66.45 2.67,70.18 3.89,71.4 SW1.1
TEMPO  (via drill 0.3)
  Top 0.152: v27.89,53.57 v27.89,37.64
  Bottom 0.152: v27.89,37.64 24.46,34.21 19.51,34.21 17.98,35.74 17.53,35.74 U1.19 | v27.89,53.57 24.69,53.57 23.77,54.48 23.77,55.32 22.94,56.16 22.1,56.16 21.26,57 21.26,59.13 20.19,60.2 POT4.2
VCC  (via drill 0.3)
  Top 0.305: v16.23,17.07 16.23,23.01 v15.24,24 15.39,24 16.69,25.3 16.69,36.8 13.72,39.78 13.72,61.87 14.71,62.87 | 14.71,62.87 v16.54,62.87 | 14.71,62.87 13.11,64.47 8,64.47 7.7,64.77 4.88,64.77 1.29,61.19 1.29,54.94 JP1.3
  Bottom 0.305: v16.23,17.07 16.23,13.03 IC4.3 | v15.24,24 14.02,25.22 14.02,26.14 C7.+ | v16.54,62.87 D1.-
VEE  (via drill 0.3)
  Top 0.305: v22.86,62.87 v27.58,62.87
  Bottom 0.305: v27.58,62.87 27.81,62.64 29.18,62.64 30.18,61.65 30.33,61.65 R37.1 | D2.+ v22.86,62.87
X_CV  (via drill 0.3)
  Top 0.152: v11.73,31.17 11.73,35.97 8.38,39.32 8.38,41 6.63,42.75 6.25,42.75 5.03,43.97 5.03,53.34 4.72,53.65 v4.72,63.55 | v16.46,83.9 v16.46,85.27
  Bottom 0.152: 16.46,84.28 18.06,84.28 R18.2 | 16.46,84.28 9.91,84.28 C1.2 9.83,84.2 9.68,84.05 9.68,79.63 7.92,77.88 6.4,77.88 2.36,73.84 2.36,66.29 4.72,63.93 v4.72,63.55 | v11.73,31.17 13.56,32.99 13.56,33.22 14.25,33.91 14.48,33.91 14.86,33.53 15.16,33.53 U1.23 | v16.46,85.27 15.62,86.11 IC1.1 | 16.46,84.28 v16.46,83.9
Y_CV  (via drill 0.3)
  Top 0.152: v12.42,30.48 12.42,35.74 9.68,38.48 9.68,60.88 9.98,61.19 9.98,62.79 v9.14,63.63 | v9.14,65.23 8,65.23 0.91,72.31 0.91,88.77 v2.44,90.3
  Bottom 0.152: C2.2 9.83,92.96 7.32,92.96 R19.2 7.24,92.89 6.48,92.13 | v12.42,30.48 14.63,32.69 14.63,32.92 U1.24 | v9.14,65.23 v9.14,63.63 | v2.44,90.3 4.27,92.13 6.48,92.13 | 6.48,92.13 6.48,90.6 6.63,90.45 9.68,90.45 10.67,89.46 13.11,89.46 14.25,90.6 14.25,90.98 IC1.7

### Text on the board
bPlace: V1.0 | PCB AND PANEL DESIGN / BY DAVID SZEBENYI / / ORIGINAL DESIGN BY / ÉMILIE GILLET / (MUTABLE INSTRUMENTS) / CC-BY-SA | ANTUMBRA | GRID | ON | JACK LIGHTS | OFF | +5V | GND | GND | CLOCK | RAND / GATE | WWW.ANTUMBRA.EU
tNames: cc-by-sa Émilie Gillet | 2014, v0.2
